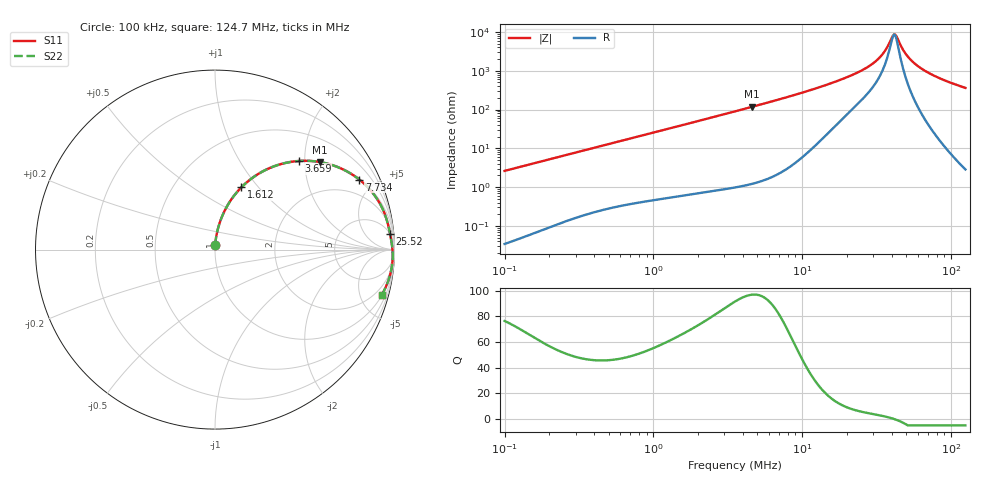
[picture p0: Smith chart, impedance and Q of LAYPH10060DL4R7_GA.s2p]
! LAYPH10060DL4R7_GA  S-PARAMETER MODEL  ( General Type )
! Model Generated by TAIYO YUDEN Corporation (http://www.ty-top.com)
! Version 3.0
! TAIYO YUDEN Control No. 180828NI43SB-FBB
! Copyright(c) 2017 TAIYO YUDEN CO.,LTD. All Rights Reserved.
! Product Description (link to TY-COMPAS)
! https://ds.yuden.co.jp/TYCOMPAS/or/detail?pn=LAYPH10060DL4R7NGA&u=M
! Products Name : Inductors
! Characteristics :
!  Inductance : 4.7 uH , SRF(min) : -Hz , DC Resistance(max) : 0.014 Ohm
!  Rated Current : Saturation :5.8 A , Temp Rise : 4.2 A (25 degC)
!  Case Size : 10.1 x 10.0 / 0.398 x 0.394 [mm/inch] , Thickness : 6 / 0.236 [mm/inch]
!  (Conditions: Temperature = 25 degC , DC Bias Current/Voltage = 0A / 0V)
! External Node Assignments :
!  1  o---GGG---o  2
! GND o---------o GND
! Frequency Range : 0.1MHz  -  124.6553MHz  [ 402 STEP ]
# MHz S RI R 50
! Freq[MHz].  S11 Real  S11 Imag  S21 Real  S21 Imag  S12 Real  S12 Imag  S22 Real  S22 Imag
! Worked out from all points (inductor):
!   401 points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, 100 kHz to 124.7 MHz, reference 50 ohm
!   read as one part in series: L = 4.18 uH near 103.6 kHz
!   highest Q = 96.9 at 4.613 MHz (marker M1), where L = 4.08 uH
!   self-resonance near 41.29 MHz
!   S11 on the Smith chart (normalised r, x): 100 kHz: 1.00, +0.05; 1.612 MHz: 1.01, +0.82; 3.659 MHz: 1.02, +1.87; 7.734 MHz: 1.06, +4.09; 25.52 MHz: 5, +21; 124.7 MHz: 1.06, -7.26
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0.1  0.00103 0.0263  0.999 -0.0263  0.999 -0.0263  0.00103 0.0263
0.330013  0.00906 0.0848  0.9909 -0.0848  0.9909 -0.0848  0.00906 0.0848
1.089088  0.0753 0.2553  0.9247 -0.2553  0.9247 -0.2553  0.0753 0.2553
1.61186  0.1473 0.3471  0.8527 -0.3471  0.8527 -0.3471  0.1473 0.3471
2.34343  0.2642 0.4345  0.7358 -0.4345  0.7358 -0.4345  0.2642 0.4345
3.530656  0.4478 0.4918  0.5522 -0.4918  0.5522 -0.4918  0.4478 0.4918
3.65876  0.4656 0.4934  0.5344 -0.4934  0.5344 -0.4934  0.4656 0.4934
4.612587  0.5823 0.4881  0.4177 -0.4881  0.4177 -0.4881  0.5823 0.4881
7.733633  0.804 0.3901  0.196 -0.3901  0.196 -0.3901  0.804 0.3901
11.65164  0.9082 0.274  0.0918 -0.274  0.0918 -0.274  0.9082 0.274
18.19151  0.9591 0.1585  0.0409 -0.1585  0.0409 -0.1585  0.9591 0.1585
25.52202  0.9752 0.089  0.0248 -0.089  0.0248 -0.089  0.9752 0.089
32.75405  0.9833 0.0435  0.0167 -0.0435  0.0167 -0.0435  0.9833 0.0435
35.80646  0.9857 0.0272  0.0143 -0.0272  0.0143 -0.0272  0.9857 0.0272
38.45196  0.9873 0.0141  0.0127 -0.0141  0.0127 -0.0141  0.9873 0.0141
40.56358  0.9883 0.00402  0.0117 -0.00402  0.0117 -0.00402  0.9883 0.00402
42.03537  0.9888 -0.00275  0.0112 0.00275  0.0112 0.00275  0.9888 -0.00275
43.56056  0.9893 -0.00959  0.0107 0.00959  0.0107 0.00959  0.9893 -0.00959
50.23514  0.9899 -0.0377  0.0101 0.0377  0.0101 0.0377  0.9899 -0.0377
60.03443  0.9878 -0.0748  0.0122 0.0748  0.0122 0.0748  0.9878 -0.0748
81.27708  0.9748 -0.1436  0.0252 0.1436  0.0252 0.1436  0.9748 -0.1436
124.6553  0.9278 -0.255  0.0722 0.255  0.0722 0.255  0.9278 -0.255
